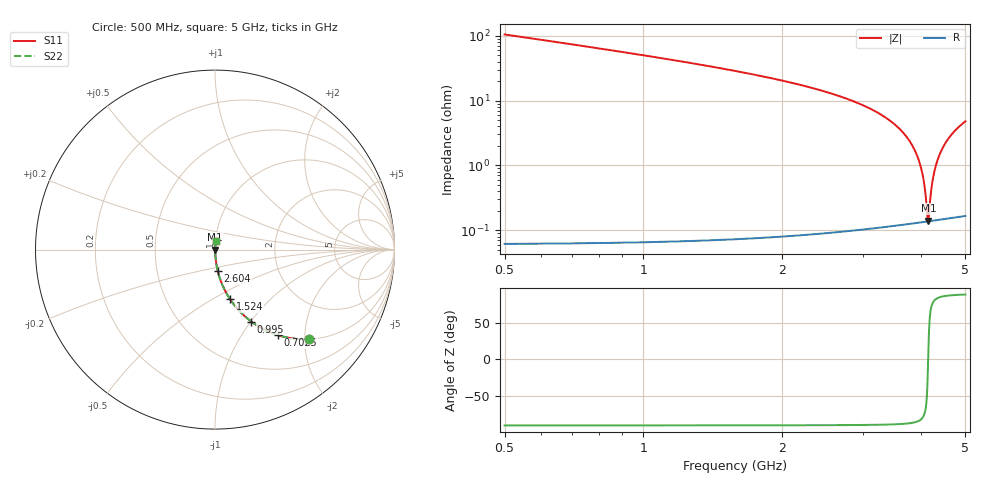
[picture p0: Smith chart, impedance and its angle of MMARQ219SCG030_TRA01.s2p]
! MMARQ219SCG030_TRA01  S-PARAMETER MODEL  ( General Type )
! Model Generated by TAIYO YUDEN Corporation (http://www.ty-top.com)
! Version 1.0
! TAIYO YUDEN Control No. 180601
! Copyright(c) 2018 TAIYO YUDEN CO.,LTD. All Rights Reserved.
! Product Description (link to TY-COMPAS)
! https://ds.yuden.co.jp/TYCOMPAS/or/detail?pn=MMARQ219SCG030BTRA01&u=M
! Products Name : Multilayer Ceramic Capacitors
! Characteristics :
!  Capacitance : 3 pF , Rated Voltage : 250V , TCC : CG / C0G
!  Case Size : 2.0 x 1.25 / 0.079 x 0.049 [mm/inch] , Thickness : 0.85 / 0.033 [mm/inch]
!  (Conditions: Temperature = 25 degC , DC Bias Current/Voltage = 0A / 0V)
! External Node Assignments :
!  1  o---| |---o  2
! GND o---------o GND
! Frequency Range : 500MHz  -  5000MHz  [ 401 STEP ]
# MHz S RI R 50
! Freq[MHz].  S11 Real  S11 Imag  S21 Real  S21 Imag  S12 Real  S12 Imag  S22 Real  S22 Imag
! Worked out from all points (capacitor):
!   401 points, 500 MHz to 5 GHz, reference 50 ohm
!   read as one part in series: C = 3 pF near 522.5 MHz
!   lowest |Z| = 141 mohm at 4.156 GHz (marker M1)
!   series resonance near 4.151 GHz, so ESL is about 490 pH
!   S11 on the Smith chart (normalised r, x): 500 MHz: 1.00, -2.09; 702.5 MHz: 1.00, -1.47; 995 MHz: 1.00, -1.00; 1.524 GHz: 1.00, -0.60; 2.604 GHz: 1.00, -0.25; 5 GHz: 1.00, +0.10
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500  0.5222 -0.4992  0.4778 0.4992  0.4778 0.4992  0.5222 -0.4992
702.5  0.3498 -0.4765  0.6502 0.4765  0.6502 0.4765  0.3498 -0.4765
995  0.2018 -0.4007  0.7982 0.4007  0.7982 0.4007  0.2018 -0.4007
1253.75  0.1292 -0.3345  0.8708 0.3345  0.8708 0.3345  0.1292 -0.3345
1523.75  0.0837 -0.2757  0.9163 0.2757  0.9163 0.2757  0.0837 -0.2757
2007.5  0.04 -0.1941  0.96 0.1941  0.96 0.1941  0.04 -0.1941
2603.75  0.0159 -0.1214  0.9841 0.1214  0.9841 0.1214  0.0159 -0.1214
2750  0.0125 -0.1067  0.9875 0.1067  0.9875 0.1067  0.0125 -0.1067
3503.75  0.00304 -0.0433  0.997 0.0433  0.997 0.0433  0.00304 -0.0433
3762.5  0.00187 -0.025  0.9981 0.025  0.9981 0.025  0.00187 -0.025
3942.5  0.00147 -0.0131  0.9985 0.0131  0.9985 0.0131  0.00147 -0.0131
4043.75  0.00138 -0.00665  0.9986 0.00665  0.9986 0.00665  0.00138 -0.00665
4088.75  0.00136 -0.00384  0.9986 0.00384  0.9986 0.00384  0.00136 -0.00384
4133.75  0.00136 -0.00105  0.9986 0.00105  0.9986 0.00105  0.00136 -0.00105
4156.25  0.00137 0.000329  0.9986 -0.000329  0.9986 -0.000329  0.00137 0.000329
4167.5  0.00137 0.00102  0.9986 -0.00102  0.9986 -0.00102  0.00137 0.00102
4223.75  0.00141 0.00443  0.9986 -0.00443  0.9986 -0.00443  0.00141 0.00443
4257.5  0.00144 0.00645  0.9986 -0.00645  0.9986 -0.00645  0.00144 0.00645
4358.75  0.00159 0.0124  0.9984 -0.0124  0.9984 -0.0124  0.00159 0.0124
4516.25  0.00195 0.0215  0.998 -0.0215  0.998 -0.0215  0.00195 0.0215
4730  0.00267 0.0333  0.9973 -0.0333  0.9973 -0.0333  0.00267 0.0333
5000  0.00392 0.0474  0.9961 -0.0474  0.9961 -0.0474  0.00392 0.0474
